PROGRAM MAIN
VAR
	bRecipe:			BOOL;//测试用的变量
	nRecipe:			INT;//测试用的变量
	rRecipe:			REAL;//测试用的变量
	lrRecipe:			LREAL;//测试用的变量
	aRecipe:			ARRAY[1..10] OF INT;//测试用的变量
	sRecipe:			STRING;	//测试用的变量
	TON_Recipe:			TON;//测试用的变量
END_VAR



SWProducts();

END_PROGRAM
